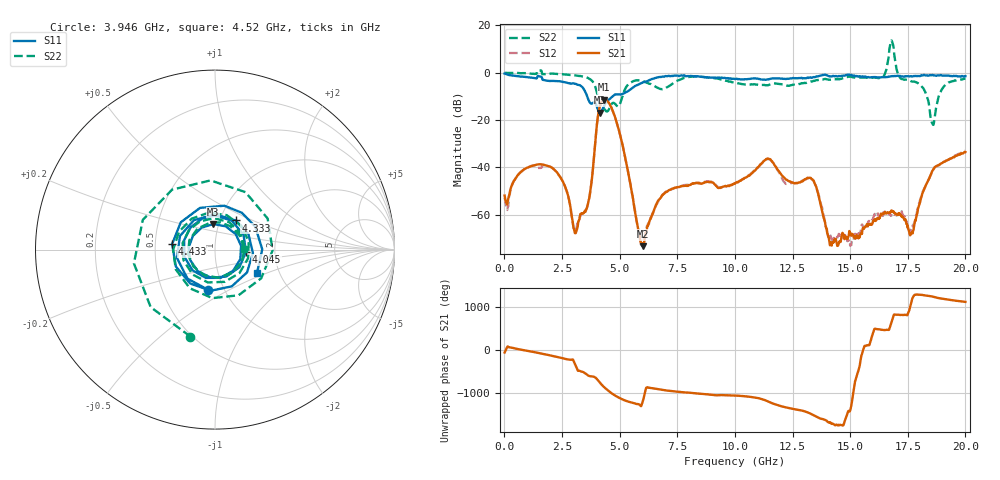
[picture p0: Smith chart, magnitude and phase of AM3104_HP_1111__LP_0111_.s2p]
!Created with skrf (http://scikit-rf.org).
# Hz S RI R 50.0
!freq ReS11 ImS11 ReS21 ImS21 ReS12 ImS12 ReS22 ImS22
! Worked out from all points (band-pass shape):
!   1601 points, 10 MHz to 20 GHz, reference 50 ohm
!   highest |S21| = -11.39 dB at 4.333 GHz (marker M1); lowest = -73.3 dB at 5.995 GHz (marker M2)
!   |S21| within 3 dB of the highest: 4.133 GHz to 4.63 GHz (496.1 MHz wide, 11.3 % of centre)
!   lowest |S11| = -16.9 dB at 4.158 GHz (marker M3), VSWR 1.33, Z = 47.1 + j13.7 ohm
!   |S11| at or under -10 dB: 3.593 GHz to 4.69 GHz (1.096 GHz wide, 26.5 % of centre)
!   |S22| runs from -22.0 to 13.6 dB; largest |S21 - S12| = 0.023
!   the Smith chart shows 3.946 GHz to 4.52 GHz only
!   S11 on the Smith chart (normalised r, x): 3.946 GHz: 0.84, -0.40; 4.045 GHz: 1.42, -0.04; 4.333 GHz: 1.18, +0.40; 4.433 GHz: 0.61, +0.04; 4.52 GHz: 1.54, -0.43
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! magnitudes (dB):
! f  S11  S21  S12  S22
! 10 MHz  -0.4  -51.9  -52.8  0.0
! 1.784 GHz  -3.2  -39.1  -39.1  -0.5
! 2.559 GHz  -3.9  -46.4  -46.5  -0.7
! 3.058 GHz  -4.7  -67.8  -66.0  -1.1
! 3.346 GHz  -5.8  -59.5  -59.6  -1.5
! 3.671 GHz  -11.9  -53.5  -53.4  -2.5
! 3.946 GHz  -12.8  -29.0  -29.0  -6.0
! 4.045 GHz  -15.2  -19.3  -19.3  -9.9
! 4.158 GHz  -16.9  -13.5  -13.6  -13.6
! 4.333 GHz  -14.0  -11.4  -11.4  -15.3
! 4.433 GHz  -12.4  -11.7  -11.8  -16.3
! 4.52 GHz  -11.5  -12.5  -12.6  -15.8
! 5.995 GHz  -4.1  -73.3  -72.6  -3.5
! 6.682 GHz  -1.9  -54.0  -54.2  -6.5
! 10.01 GHz  -2.7  -46.9  -46.9  -4.3
! 11.44 GHz  -2.8  -36.3  -36.4  -5.3
! 13.34 GHz  -2.1  -45.0  -44.9  -3.7
! 14.19 GHz  -1.5  -72.5  -70.1  -2.9
! 16.68 GHz  -1.6  -59.2  -59.8  7.2
! 17.66 GHz  -1.6  -67.6  -67.5  -3.7
! 18.58 GHz  -1.0  -41.3  -41.7  -21.6
! 20 GHz  -1.4  -33.5  -33.0  -2.5
